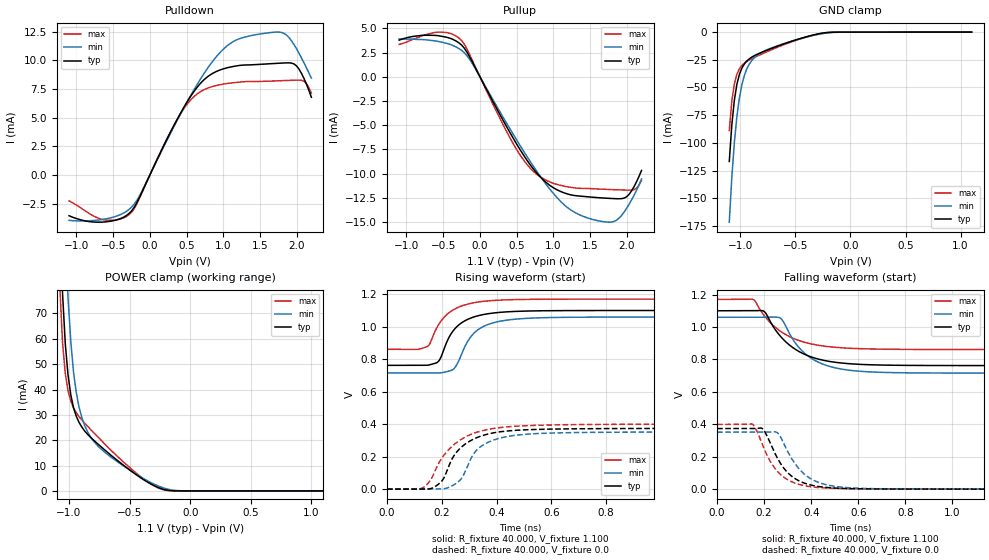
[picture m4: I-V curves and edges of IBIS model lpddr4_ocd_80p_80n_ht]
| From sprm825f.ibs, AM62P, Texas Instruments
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|   Model lpddr4_ocd_80p_80n_ht
[Model] lpddr4_ocd_80p_80n_ht
Model_type I/O
Polarity   Non-Inverting
Enable   Active-High
Vinl =  0.113V
Vinh =  0.253V
Vmeas =  0.183V
C_comp   2.560pF   2.545pF   2.583pF
[Model Spec]
Vinh   0.253V   0.247V   0.265V
Vinl   0.113V   0.107V   0.125V
Vmeas   0.183V   0.176V   0.195V
[Temperature Range]   25.000   0.125k   -40.000
[Voltage Range]   1.100V   1.060V   1.170V
[Pullup Reference]   1.100V   1.060V   1.170V
[Pulldown Reference]   0.0V   0.0V   0.0V
[C Comp Corner]
C_comp   2.560pF   2.545pF   2.583pF
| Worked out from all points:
|   slope of the pulldown table from 0 to 0.165 V, typ, clamps not added: 73.9 ohm
|   slope of the pullup table from 0 to 0.165 V, typ, clamps not added: 69 ohm
|   GND clamp passes 1 mA (typ) near -0.26 V on its own axis
|   POWER clamp passes 1 mA (typ) near -0.24 V on its own axis
|   rising waveform, R_fixture 40.000, V_fixture 1.100: 20-80 % time 79ps typ, 80.4ps min, 83.4ps max; typ from 0.762 V to 1.1 V
|   rising waveform, R_fixture 40.000, V_fixture 0.0: 20-80 % time 96.6ps typ, 87.7ps min, 118ps max; typ from 0.001 V to 0.375 V
|   falling waveform, R_fixture 40.000, V_fixture 1.100: 20-80 % time 148ps typ, 132ps min, 154ps max; typ from 1.1 V to 0.762 V
|   falling waveform, R_fixture 40.000, V_fixture 0.0: 20-80 % time 100ps typ, 108ps min, 96.9ps max; typ from 0.374 V to 0.001 V
[Pulldown]
|Voltage   I(typ)   I(min)   I(max)
-1.1V     -3.54mA    -3.942mA   -2.243mA
-624mV    -4.087mA   -3.846mA   -3.891mA
-284mV    -3.349mA   -2.996mA   -3.451mA
-147mV    -2.034mA   -1.882mA   -2.101mA
261mV     3.483mA    3.384mA    3.52mA
533mV     6.638mA    6.672mA    6.384mA
805mV     8.66mA     9.483mA    7.621mA
1.145V    9.481mA    11.67mA    8.057mA
1.826V    9.773mA    12.36mA    8.238mA
1.996V    9.529mA    11.03mA    8.278mA
2.098V    8.441mA    9.8mA      8.195mA
2.2V      6.782mA    8.453mA    7.144mA
[Pullup]
|Voltage   I(typ)   I(min)   I(max)
-1.1V     3.776mA    3.904mA    3.339mA
-590mV    4.258mA    3.678mA    4.595mA
-284mV    3.487mA    2.901mA    3.984mA
-113mV    1.667mA    1.486mA    1.855mA
329mV     -4.692mA   -4.361mA   -5.163mA
601mV     -8.178mA   -7.767mA   -8.672mA
907mV     -10.96mA   -11.17mA   -10.72mA
1.281V    -12.27mA   -13.97mA   -11.48mA
1.826V    -12.59mA   -14.95mA   -11.67mA
2.03V     -12.16mA   -13.19mA   -11.72mA
2.132V    -10.86mA   -11.73mA   -11.52mA
2.2V      -9.689mA   -10.57mA   -10.71mA
[GND_clamp]
|Voltage   I(typ)   I(min)   I(max)
-1.1V     -116.8mA   -171.6mA   -88.94mA
-1.077V   -83.96mA   -131.3mA   -62.39mA
-1.054V   -61.6mA    -99.87mA   -46.82mA
-1.031V   -47.19mA   -76.34mA   -38.11mA
-1.008V   -38.16mA   -59.32mA   -33.12mA
-985mV    -32.43mA   -47.3mA    -30.04mA
-940mV    -26mA      -32.95mA   -26.37mA
-894mV    -22.48mA   -25.52mA   -23.91mA
-848mV    -20.08mA   -21.13mA   -21.75mA
-619mV    -11.17mA   -10.91mA   -11.97mA
-229mV    -598.7uA   -1.001mA   -573.1uA
1.1V      0A         0A         0A
[POWER_clamp]
|Voltage   I(typ)   I(min)   I(max)
-1.1V     158.5mA    248.7mA    122.8mA
-1.077V   110.5mA    184.5mA    81.81mA
-1.054V   78.43mA    136mA      58.82mA
-1.031V   58.13mA    100.8mA    46.37mA
-1.008V   45.61mA    75.97mA    39.54mA
-985mV    37.81mA    58.74mA    35.43mA
-963mV    32.84mA    46.93mA    32.78mA
-940mV    29.44mA    38.74mA    30.8mA
-871mV    23.65mA    25.79mA    26.71mA
-642mV    13.62mA    12.94mA    15.51mA
-206mV    448.9uA    953.4uA    285.6uA
1.1V      0A         0A         0A
[Ramp]
| variable   typ   min   max
dV/dt_r   0.224/96.443p   0.211/87.418p   0.239/0.118n
dV/dt_f   0.203/0.148n   0.207/0.132n   0.185/0.154n
R_load = 40.000
[Rising Waveform]
R_fixture= 40.000
V_fixture= 1.100
V_fixture_min= 1.060
V_fixture_max= 1.170
|time   V(typ)   V(min)   V(max)
0s        762.3mV    715.6mV    861mV
145ps     762.3mV    715.7mV    876.5mV
181ps     778.2mV    715.2mV    991.1mV
234ps     956.4mV    731mV      1.095V
254ps     998.4mV    763.7mV    1.115V
301ps     1.05V      926.2mV    1.142V
339ps     1.07V      988.9mV    1.153V
413ps     1.088V     1.034V     1.164V
535ps     1.097V     1.053V     1.168V
5ns       1.1V       1.06V      1.17V
[Rising Waveform]
R_fixture= 40.000
V_fixture= 0.0
V_fixture_min= 0.0
V_fixture_max= 0.0
|time   V(typ)   V(min)   V(max)
0s        1.128mV    1.69mV     2.398mV
134ps     1.048mV    1.683mV    12.73mV
161ps     5.3mV      1.675mV    62.98mV
195ps     41.87mV    1.726mV    178.7mV
225ps     140.4mV    11.36mV    243.6mV
269ps     255.4mV    60.64mV    305.2mV
313ps     306.3mV    208.7mV    342.4mV
345ps     328.6mV    265.9mV    359.5mV
501ps     365.8mV    337.8mV    390.7mV
5ns       374.9mV    353.2mV    400.5mV
[Falling Waveform]
R_fixture= 40.000
V_fixture= 1.100
V_fixture_min= 1.060
V_fixture_max= 1.170
|time   V(typ)   V(min)   V(max)
0s        1.1V       1.06V      1.17V
154ps     1.1V       1.06V      1.169V
202ps     1.093V     1.06V      1.067V
264ps     951.6mV    1.058V     979.2mV
280ps     925.5mV    1.037V     963.4mV
342ps     854mV      883.9mV    919.6mV
409ps     811.2mV    799.6mV    893mV
506ps     781.9mV    747.1mV    874.3mV
653ps     767.2mV    723.1mV    864.6mV
5ns       762.3mV    715.6mV    861mV
[Falling Waveform]
R_fixture= 40.000
V_fixture= 0.0
V_fixture_min= 0.0
V_fixture_max= 0.0
|time   V(typ)   V(min)   V(max)
0s        374.4mV    352.1mV    400.1mV
151ps     374.2mV    352.1mV    401mV
196ps     368.9mV    352mV      263.3mV
253ps     201.3mV    351.4mV    116.2mV
298ps     106.1mV    238.9mV    61.02mV
353ps     49.07mV    118.8mV    28.67mV
399ps     26.46mV    64.64mV    16.05mV
458ps     12.61mV    30.63mV    8.507mV
782ps     1.84mV     2.704mV    2.769mV
5ns       1.127mV    1.68mV     2.399mV
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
